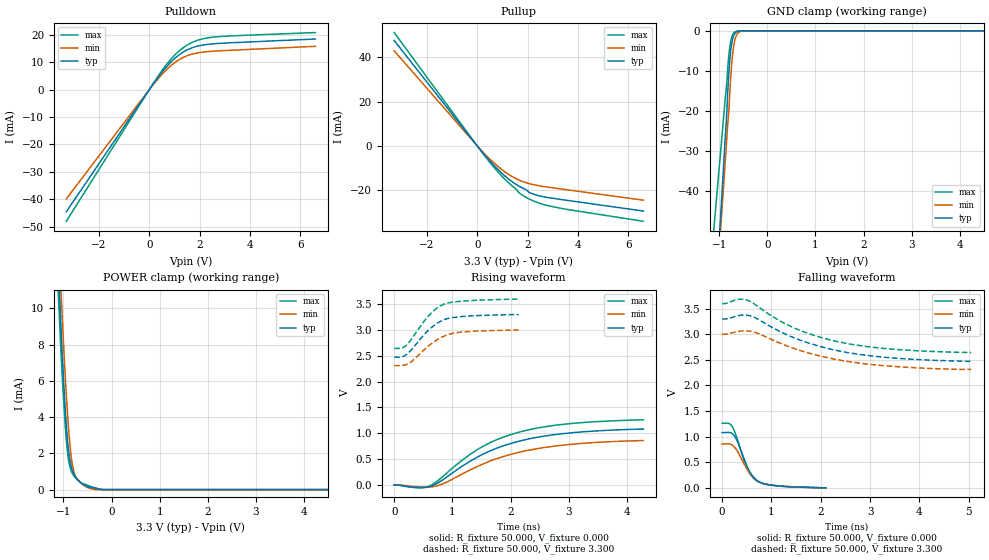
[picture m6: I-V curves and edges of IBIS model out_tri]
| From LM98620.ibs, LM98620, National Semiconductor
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[Model]   out_tri
Model_type 3-state
Vref=0.000E+00
Rref=1.000E+06
Cref=0.000E+00
Vmeas=1.650E+00
C_comp   1.130E-12   1.000E-12   1.220E-12
[Voltage Range]   3.300E+00   3.000E+00   3.600E+00
[POWER Clamp Reference]   3.300E+00   3.000E+00   3.600E+00
[GND Clamp Reference]   0.000E+00   0.000E+00   0.000E+00
[Pullup Reference]   3.300E+00   3.000E+00   3.600E+00
[Pulldown Reference]   0.000E+00   0.000E+00   0.000E+00
[Temperature Range]   25   70   0
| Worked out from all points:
|   slope of the pulldown table from 0 to 0.495 V, typ, clamps not added: 79.5 ohm
|   slope of the pullup table from 0 to 0.495 V, typ, clamps not added: 74.2 ohm
|   GND clamp passes 1 mA (typ) near -0.69 V on its own axis
|   POWER clamp passes 1 mA (typ) near -0.81 V on its own axis
|   rising waveform, R_fixture 50.000, V_fixture 0.000: 20-80 % time 1.23ns typ, 1.28ns min, 1.18ns max; typ from 0 V to 1.08 V
|   falling waveform, R_fixture 50.000, V_fixture 0.000: 20-80 % time 303ps typ, 340ps min, 294ps max; typ from 1.08 V to 0 V
|   rising waveform, R_fixture 50.000, V_fixture 3.300: 20-80 % time 430ps typ, 463ps min, 412ps max; typ from 2.47 V to 3.3 V
|   falling waveform, R_fixture 50.000, V_fixture 3.300: 20-80 % time 1.55ns typ, 1.6ns min, 1.52ns max; typ from 3.3 V to 2.47 V
[GND Clamp]
-3.3V     -521.8mA   -464.1mA   -350mA
-900mV    -31.48mA   -36.89mA   -20.26mA
-860mV    -23.82mA   -29.77mA   -15.17mA
-800mV    -10.29mA   -19.8mA    -5.923mA
-780mV    -7.073mA   -15.2mA    -3.863mA
-760mV    -4.718mA   -11.23mA   -2.438mA
-720mV    -1.924mA   -5.581mA   -877.2uA
-700mV    -1.191mA   -3.78mA    -507.6uA
-660mV    -461.7uA   -1.659mA   -181uA
-600mV    -115.6uA   -436.9uA   -45.85uA
-500mV    0A         0A         0A
6.6V      0A         0A         0A
[Power Clamp]
-3.3V     142.4mA    142.1mA    131.9mA
-1.12V    13.08mA    15.04mA    11.46mA
-1.1V     11.92mA    13.9mA     10.42mA
-1.06V    9.477mA    11.5mA     8.064mA
-1.04V    8.3mA      10.36mA    6.988mA
-980mV    5.198mA    7.117mA    4.224mA
-940mV    3.533mA    5.222mA    2.725mA
-880mV    1.867mA    2.926mA    1.425mA
-820mV    1.09mA     1.456mA    913.9uA
-720mV    597.3uA    601.3uA    559.5uA
-480mV    141.8uA    95.45uA    218.5uA
6.6V      0A         0A         0A
[Pullup]
-3.3V     47.47mA    42.83mA    51.06mA
0V        0A         0A         0A
340mV     -4.697mA   -4.096mA   -5.083mA
760mV     -9.908mA   -8.593mA   -10.87mA
1.06V     -13.11mA   -11.31mA   -14.55mA
1.42V     -16.34mA   -13.99mA   -18.29mA
1.7V      -18.36mA   -15.53mA   -21.4mA
1.96V     -19.85mA   -16.59mA   -23.27mA
2.08V     -21.03mA   -16.98mA   -23.95mA
2.46V     -22.45mA   -17.92mA   -25.73mA
2.86V     -23.3mA    -18.62mA   -27.01mA
6.6V      -29.28mA   -24.39mA   -33.9mA
[Pulldown]
-3.3V     -44.48mA   -39.8mA    -47.95mA
160mV     2.127mA    1.863mA    2.315mA
500mV     6.287mA    5.488mA    6.877mA
800mV     9.449mA    8.201mA    10.4mA
1.04V     11.57mA    9.987mA    12.81mA
1.3V      13.36mA    11.45mA    14.89mA
1.74V     15.32mA    12.97mA    17.3mA
1.96V     15.88mA    13.38mA    18.05mA
2.42V     16.53mA    13.86mA    18.92mA
3.32V     17.04mA    14.31mA    19.55mA
6.6V      18.38mA    15.72mA    20.72mA
[Rising Waveform]
R_fixture = 50.000
V_fixture = 0.000
V_fixture_min = 0.000
V_fixture_max = 0.000
|  time   V(typ)   V(min)   V(max)
0s        0V         0V         0V
405ps     -49.96mV   -38.48mV   -57.13mV
595ps     -38.13mV   -43.69mV   -28.36mV
880ps     131.6mV    41.06mV    203.9mV
1.145ns   344.5mV    196.6mV    457.1mV
1.44ns    543.4mV    361.6mV    691.1mV
1.785ns   719.6mV    515.7mV    885.3mV
2.19ns    858.4mV    642.8mV    1.034V
2.985ns   1.002V     779.2mV    1.182V
4.285ns   1.08V      858.3mV    1.261V
[Falling Waveform]
R_fixture = 50.000
V_fixture = 0.000
V_fixture_min = 0.000
V_fixture_max = 0.000
|  time   V(typ)   V(min)   V(max)
0s        1.08V      858.3mV    1.261V
150ps     1.082V     857.1mV    1.253V
245ps     1.022V     801.4mV    1.121V
315ps     897.2mV    708.2mV    934.2mV
500ps     434.5mV    373.3mV    395.2mV
600ps     254.7mV    235.1mV    229.9mV
705ps     146.4mV    143.1mV    134.7mV
850ps     79.25mV    78.75mV    79.77mV
1.12ns    38.47mV    37.89mV    42.22mV
2.105ns   0V         0V         0V
[Rising Waveform]
R_fixture = 50.000
V_fixture = 3.300
V_fixture_min = 3.000
V_fixture_max = 3.600
|  time   V(typ)   V(min)   V(max)
0s        2.474V     2.313V     2.645V
130ps     2.479V     2.313V     2.652V
205ps     2.521V     2.33V      2.702V
310ps     2.636V     2.401V     2.845V
605ps     3.013V     2.707V     3.293V
730ps     3.125V     2.807V     3.423V
850ps     3.199V     2.879V     3.5V
995ps     3.241V     2.933V     3.54V
1.165ns   3.263V     2.962V     3.561V
2.14ns    3.3V       3V         3.6V
[Falling Waveform]
R_fixture = 50.000
V_fixture = 3.300
V_fixture_min = 3.000
V_fixture_max = 3.600
|  time   V(typ)   V(min)   V(max)
0s        3.3V       3V         3.6V
325ps     3.364V     3.056V     3.682V
500ps     3.374V     3.066V     3.671V
705ps     3.307V     3.025V     3.557V
1.115ns   3.083V     2.85V      3.294V
1.515ns   2.909V     2.704V     3.101V
1.97ns    2.767V     2.579V     2.948V
2.47ns    2.655V     2.481V     2.831V
3.605ns   2.527V     2.363V     2.698V
5.05ns    2.474V     2.313V     2.645V
[Ramp]
dV/dt_r   6.3728E-01/1.2302E-09   5.0731E-01/1.2816E-09   7.4558E-01/1.1812E-09
dV/dt_f   4.9590E-01/1.5546E-09   4.1219E-01/1.5944E-09   5.7327E-01/1.5210E-09
R_load = 50
